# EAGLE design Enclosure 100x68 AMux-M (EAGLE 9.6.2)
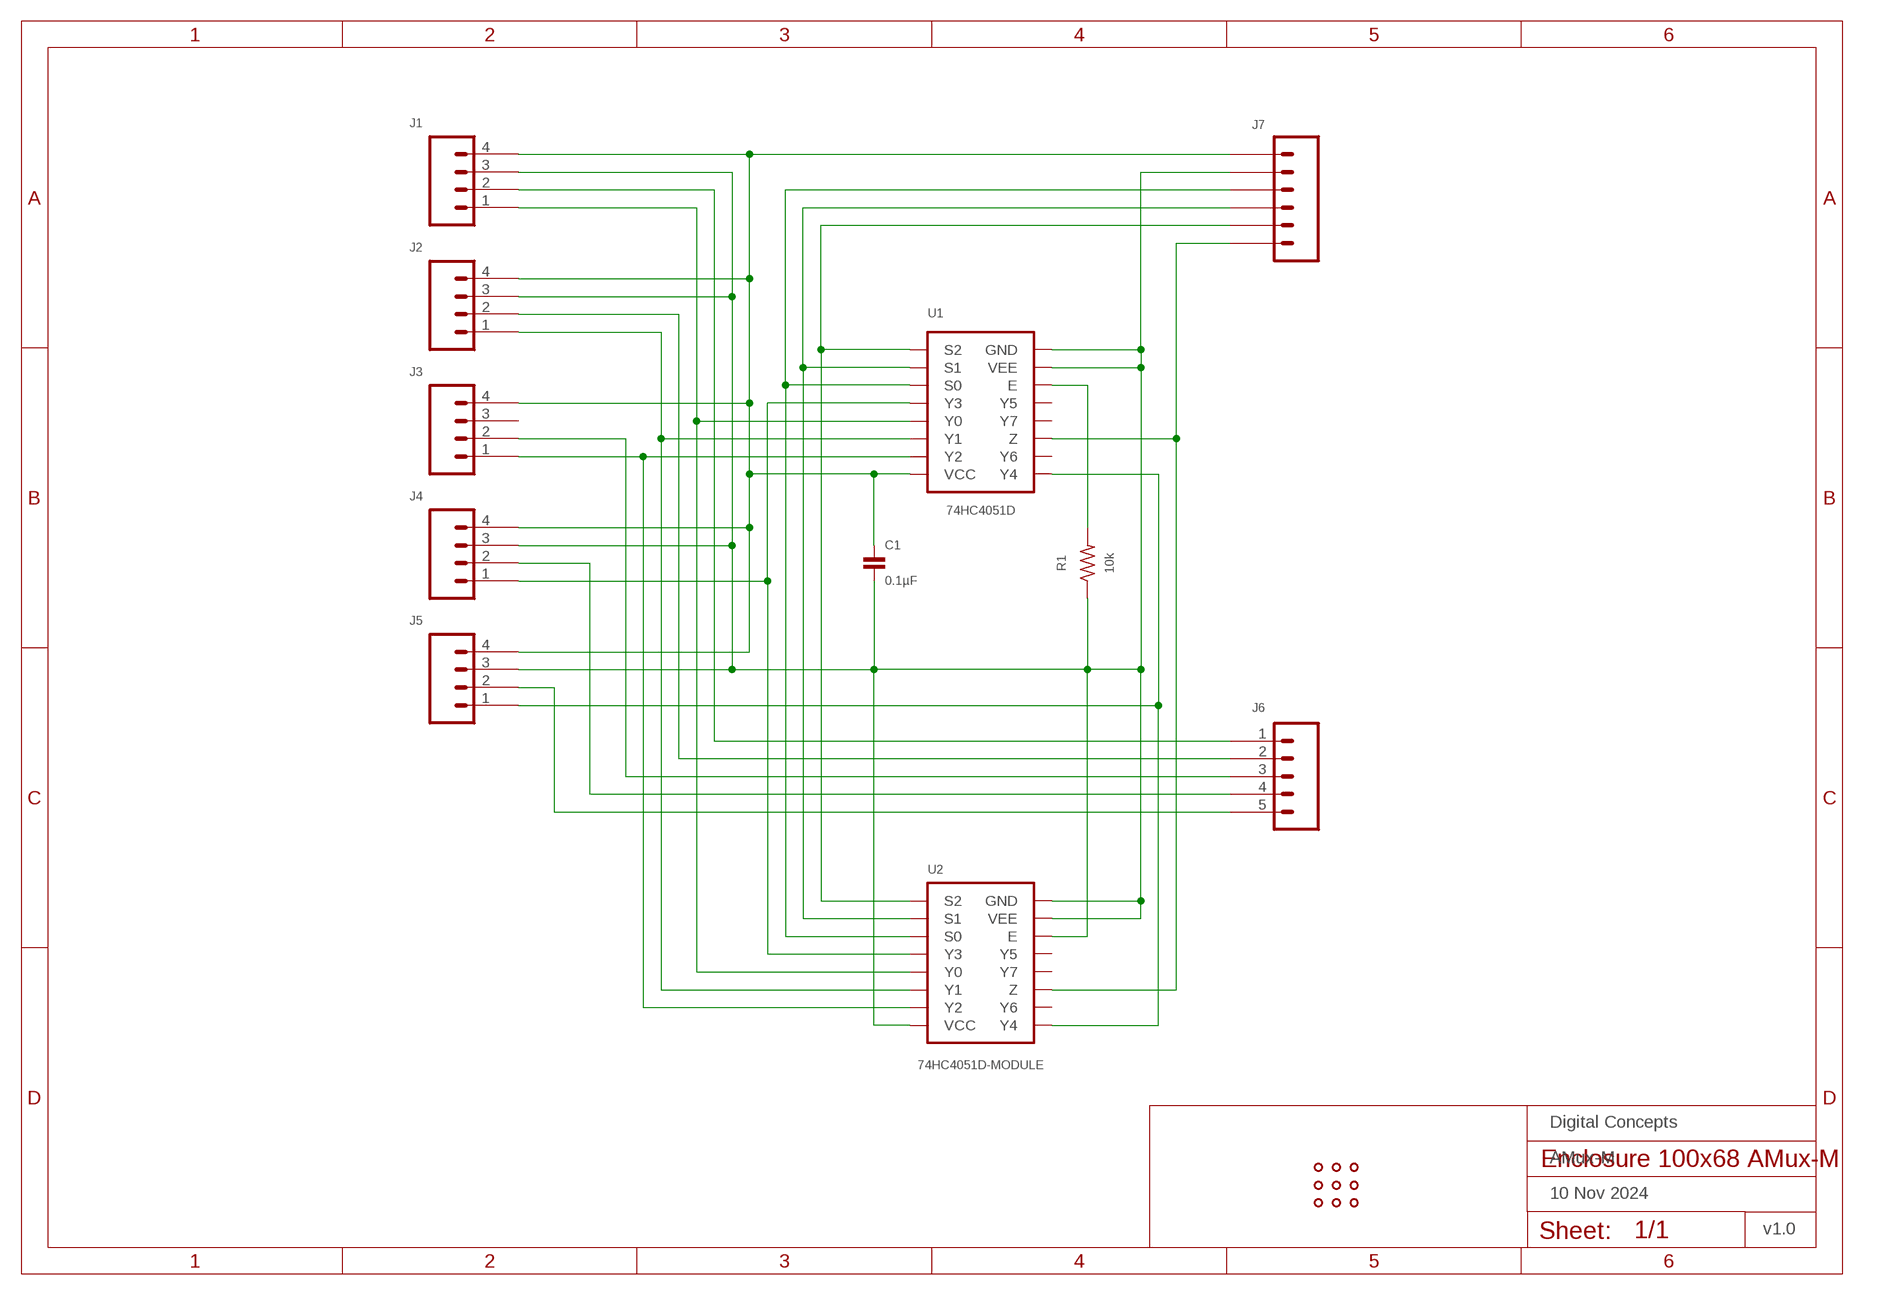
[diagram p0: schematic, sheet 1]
FRAME1 (A4L-LOC): DATE: 10 Nov 2024; OWNER: Digital Concepts; TITLE: AMux-M; VERSION: v1.0

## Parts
C1  0.1µF  CAPACITOR-0805  [C0805]
J1  HEADER-1X4-GENERIC  [CONN_04-GENERIC]
J2  HEADER-1X4-GENERIC  [CONN_04-GENERIC]
J3  HEADER-1X4-GENERIC  [CONN_04-GENERIC]
J4  HEADER-1X4-GENERIC  [CONN_04-GENERIC]
J5  HEADER-1X4-GENERIC  [CONN_04-GENERIC]
J6  JST-PH2.0-5-HORIZONTAL  [JST-PH2.0-5-HORIZONTAL]
J7  JST-PH2.0-6-HORIZONTAL  [JST-PH2.0-6-HORIZONTAL]
R1  10k  RESISTORR0805  [R0805]
U1  74HC4051D  [SOP16]
U2  74HC4051D-MODULE  [74HC4051D-MODULE]
U$1  PROTO-34X22-AMUX  [PROTO-34X22-AMUX]

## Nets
GND: C1.2 J1.3 J2.3 J4.3 J5.3 J7.2 R1.1 U1.7(VEE) U1.8(GND) U2.E U2.GND@L(GND) U2.GND@R(GND) U2.VCC@L(VCC) U2.VCC@R(VCC) U2.VEE@L(VEE) U2.VEE@R(VEE)
N$1: J4.1 U1.12(Y3) U2.Y3
N$2: J2.1 U1.14(Y1) U2.Y1
N$3: J1.1 U1.13(Y0) U2.Y0
N$4: J3.1 U1.15(Y2) U2.Y2
N$5: J5.1 U1.1(Y4) U2.Y4
N$6: J7.3 U1.11(S0) U2.S0
N$7: J7.4 U1.10(S1) U2.S1
N$8: R1.2 U1.6(E)
N$9: J7.6 U1.3(Z) U2.Z
N$13: J1.2 J6.1
N$16: J7.5 U1.9(S2) U2.S2
N$17: J2.2 J6.2
N$18: J3.2 J6.3
N$19: J4.2 J6.4
N$20: J5.2 J6.5
N$26: C1.1 J1.4 J2.4 J3.4 J4.4 J5.4 J7.1 U1.16(VCC)
Unconnected: J3.3 U1.2(Y6) U1.4(Y7) U1.5(Y5) U2.Y5 U2.Y6 U2.Y7

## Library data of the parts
C1 = digitalconcepts:CAPACITOR-0805: 0805 Capacitor
J1-J5 = digitalconcepts:HEADER-1X4-GENERIC: Single Row 4-Pin Header
J6 = digitalconcepts:JST-PH2.0-5-HORIZONTAL: PH2.0 5P Horizontal Connector
J7 = digitalconcepts:JST-PH2.0-6-HORIZONTAL: PH2.0 6P Horizontal Connector
R1 = digitalconcepts:RESISTOR: Resistor; SPICEPREFIX: R
U1 = digitalconcepts:74HC4051D: 74HC4051 8-Port Multiplexer SOP-16
U2 = digitalconcepts:74HC4051D-MODULE: 74HC4051 8-Port Analog Multiplexer Module
U$1 = digitalconcepts:PROTO-34X22-AMUX: 34 x 22 Analog Mux Prototyping board to fit an 100 x 68 enclosure

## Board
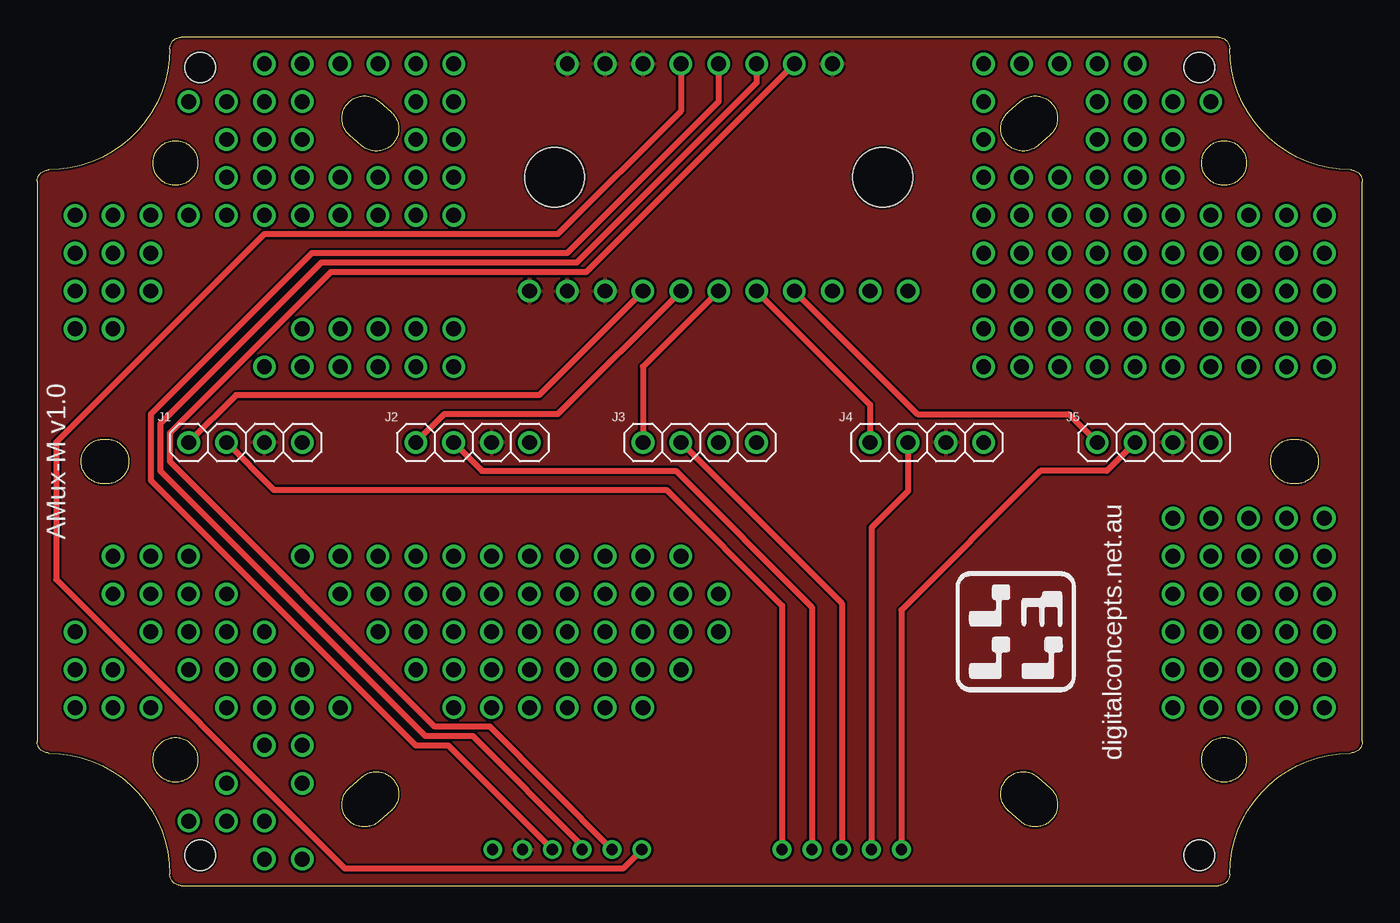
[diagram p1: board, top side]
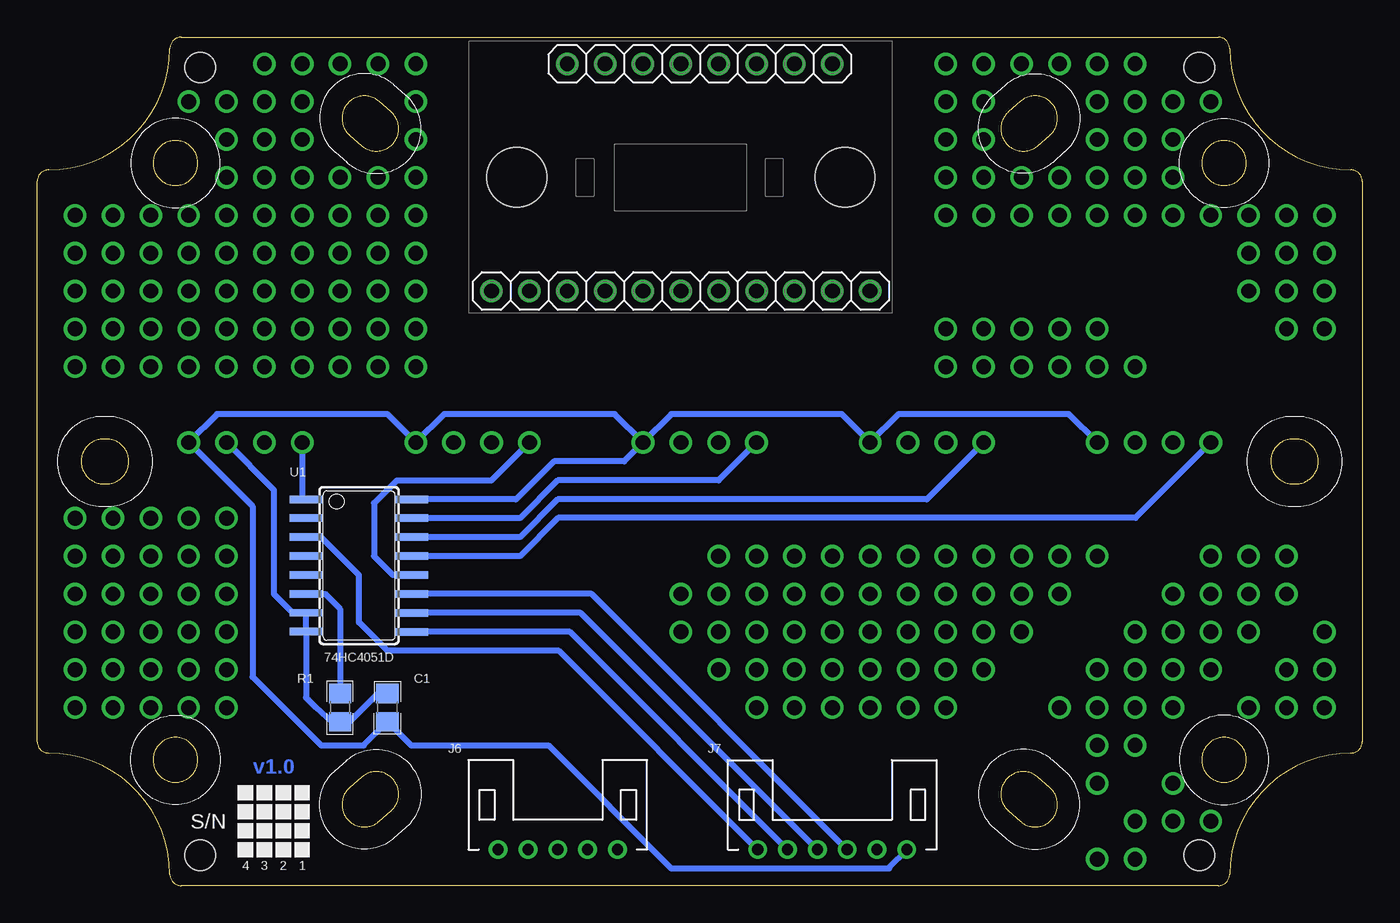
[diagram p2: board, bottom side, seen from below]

Size 88.9 x 56.9 mm. Coordinates in mm from the lower left corner, seen from the top.
Copper layers (1*16): Top 0.035mm / dielectric 1.5mm / Bottom 0.035mm
Design rules "default *": minimum track width 6mil, minimum drill 0.35mm, track to track 6mil, track to pad 6mil, pad to pad 6mil, via to via 6mil, smd to smd 6mil, copper to edge 6mil, drill to drill 6mil, minimum pad ring 10mil, minimum via ring 8mil, stop-mask expansion 4mil, vias tented up to drill 0mil, thermal gap 6mil

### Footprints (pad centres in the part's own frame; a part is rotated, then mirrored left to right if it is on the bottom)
C0805 = smd 1.3 x 1.5: 1 -0.95,0; 2 0.95,0
CONN_04-GENERIC = drill 1 pad 1.524: 1 0,0; 2 2.54,0; 3 5.08,0; 4 7.62,0
JST-PH2.0-5-HORIZONTAL = drill 0.75: 1 4,0; 2 2,0; 3 0,0; 4 -2,0; 5 -4,0
JST-PH2.0-6-HORIZONTAL = drill 0.75: 1 5,0; 2 3,0; 3 1,0; 4 -1,0; 5 -3,0; 6 -5,0
R0805 = smd 1.3 x 1.5: 1 -0.95,0; 2 0.95,0
SOP16 = smd 0.5 x 2.2: 1 -4.445,-3.55; 2 -3.185,-3.55; 3 -1.915,-3.55; 4 -0.645,-3.55; 5 0.635,-3.55; 6 1.895,-3.55; 7 3.165,-3.55; 8 4.435,-3.55; 9 4.445,3.55; 10 3.175,3.55; 11 1.905,3.55; 12 0.635,3.55; 13 -0.635,3.55; 14 -1.905,3.55; 15 -3.175,3.55; 16 -4.445,3.55
74HC4051D-MODULE = drill 1: E 0,5.08; GND@L 0,17.78; GND@R 15.24,20.32; S0 0,12.7; S1 0,10.16; S2 0,7.62; VCC@L 0,20.32; VCC@R 15.24,22.86; VEE@L 0,22.86; VEE@R 15.24,25.4; Y0 15.24,17.78; Y1 15.24,15.24; Y2 15.24,12.7; Y3 15.24,10.16; Y4 15.24,7.62; Y5 15.24,5.08; Y6 15.24,2.54; Y7 15.24,0; Z 0,15.24 | hole 4: 7.62,23.7; 7.62,1.7
PROTO-34X22-AMUX = drill 1: P01-05 -41.91,-16.51; P01-06 -41.91,-13.97; P01-07 -41.91,-11.43; P01-15 -41.91,8.89; P01-16 -41.91,11.43; P01-17 -41.91,13.97; P01-18 -41.91,16.51; P02-05 -39.37,-16.51; P02-06 -39.37,-13.97; P02-08 -39.37,-8.89; P02-09 -39.37,-6.35; P02-15 -39.37,8.89; P02-16 -39.37,11.43; P02-17 -39.37,13.97; P02-18 -39.37,16.51; P03-05 -36.83,-16.51; P03-07 -36.83,-11.43; P03-08 -36.83,-8.89; P03-09 -36.83,-6.35; P03-16 -36.83,11.43; P03-17 -36.83,13.97; P03-18 -36.83,16.51; P04-02 -34.29,-24.13; P04-06 -34.29,-13.97; P04-07 -34.29,-11.43; P04-08 -34.29,-8.89; P04-09 -34.29,-6.35; P04-18 -34.29,16.51; P04-21 -34.29,24.13; P05-02 -31.75,-24.13; P05-03 -31.75,-21.59; P05-05 -31.75,-16.51; P05-06 -31.75,-13.97; P05-07 -31.75,-11.43; P05-08 -31.75,-8.89; P05-18 -31.75,16.51; P05-19 -31.75,19.05; P05-20 -31.75,21.59; P05-21 -31.75,24.13; P06-01 -29.21,-26.67; P06-02 -29.21,-24.13; P06-04 -29.21,-19.05; P06-05 -29.21,-16.51; P06-06 -29.21,-13.97; P06-07 -29.21,-11.43; P06-14 -29.21,6.35; P06-18 -29.21,16.51; P06-19 -29.21,19.05; P06-20 -29.21,21.59; P06-21 -29.21,24.13; P06-22 -29.21,26.67; P07-01 -26.67,-26.67; P07-03 -26.67,-21.59; P07-04 -26.67,-19.05; P07-05 -26.67,-16.51; P07-06 -26.67,-13.97; P07-09 -26.67,-6.35; P07-14 -26.67,6.35; P07-15 -26.67,8.89; P07-18 -26.67,16.51; P07-19 -26.67,19.05; P07-20 -26.67,21.59; P07-21 -26.67,24.13; P07-22 -26.67,26.67; P08-05 -24.13,-16.51; P08-08 -24.13,-8.89; P08-09 -24.13,-6.35; P08-14 -24.13,6.35; P08-15 -24.13,8.89; P08-18 -24.13,16.51; P08-19 -24.13,19.05; P08-22 -24.13,26.67; P09-07 -21.59,-11.43; P09-08 -21.59,-8.89; P09-09 -21.59,-6.35; P09-14 -21.59,6.35; P09-15 -21.59,8.89; P09-18 -21.59,16.51; P09-19 -21.59,19.05; P09-22 -21.59,26.67; P10-06 -19.05,-13.97; P10-07 -19.05,-11.43; P10-08 -19.05,-8.89; P10-09 -19.05,-6.35; P10-14 -19.05,6.35; P10-15 -19.05,8.89; P10-18 -19.05,16.51; P10-19 -19.05,19.05; P10-20 -19.05,21.59; P10-21 -19.05,24.13; P10-22 -19.05,26.67; P11-05 -16.51,-16.51; P11-06 -16.51,-13.97; P11-07 -16.51,-11.43; P11-08 -16.51,-8.89; P11-09 -16.51,-6.35; P11-14 -16.51,6.35; P11-15 -16.51,8.89; P11-18 -16.51,16.51; P11-19 -16.51,19.05; P11-20 -16.51,21.59; P11-21 -16.51,24.13; P11-22 -16.51,26.67; P12-05 -13.97,-16.51; P12-06 -13.97,-13.97; P12-07 -13.97,-11.43; P12-08 -13.97,-8.89; P12-09 -13.97,-6.35; P13-05 -11.43,-16.51; P13-06 -11.43,-13.97; P13-07 -11.43,-11.43; P13-08 -11.43,-8.89; P13-09 -11.43,-6.35; P14-05 -8.89,-16.51; P14-06 -8.89,-13.97; P14-07 -8.89,-11.43; P14-08 -8.89,-8.89; P14-09 -8.89,-6.35; P15-05 -6.35,-16.51; P15-06 -6.35,-13.97; P15-07 -6.35,-11.43; P15-08 -6.35,-8.89; P15-09 -6.35,-6.35; P16-05 -3.81,-16.51; P16-06 -3.81,-13.97; P16-07 -3.81,-11.43; P16-08 -3.81,-8.89; P16-09 -3.81,-6.35; P17-06 -1.27,-13.97; P17-07 -1.27,-11.43; P17-08 -1.27,-8.89; P17-09 -1.27,-6.35; P18-07 1.27,-11.43; P18-08 1.27,-8.89; P25-14 19.05,6.35; P25-15 19.05,8.89; P25-16 19.05,11.43; P25-17 19.05,13.97; P25-18 19.05,16.51; P25-19 19.05,19.05; P25-20 19.05,21.59; P25-21 19.05,24.13; P25-22 19.05,26.67; P26-14 21.59,6.35; P26-15 21.59,8.89; P26-16 21.59,11.43; P26-17 21.59,13.97; P26-18 21.59,16.51; P26-19 21.59,19.05; P26-22 21.59,26.67; P27-14 24.13,6.35; P27-15 24.13,8.89; P27-16 24.13,11.43; P27-17 24.13,13.97; P27-18 24.13,16.51; P27-19 24.13,19.05; P27-22 24.13,26.67; P28-14 26.67,6.35; P28-15 26.67,8.89; P28-16 26.67,11.43; P28-17 26.67,13.97; P28-18 26.67,16.51; P28-19 26.67,19.05; P28-20 26.67,21.59; P28-21 26.67,24.13; P28-22 26.67,26.67; P29-14 29.21,6.35; P29-15 29.21,8.89; P29-16 29.21,11.43; P29-17 29.21,13.97; P29-18 29.21,16.51; P29-19 29.21,19.05; P29-20 29.21,21.59; P29-21 29.21,24.13; P29-22 29.21,26.67; P30-05 31.75,-16.51; P30-06 31.75,-13.97; P30-07 31.75,-11.43; P30-08 31.75,-8.89; P30-09 31.75,-6.35; P30-10 31.75,-3.81; P30-14 31.75,6.35; P30-15 31.75,8.89; P30-16 31.75,11.43; P30-17 31.75,13.97; P30-18 31.75,16.51; P30-19 31.75,19.05; P30-20 31.75,21.59; P30-21 31.75,24.13; P31-05 34.29,-16.51; P31-06 34.29,-13.97; P31-07 34.29,-11.43; P31-08 34.29,-8.89; P31-09 34.29,-6.35; P31-10 34.29,-3.81; P31-14 34.29,6.35; P31-15 34.29,8.89; P31-16 34.29,11.43; P31-17 34.29,13.97; P31-18 34.29,16.51; P31-21 34.29,24.13; P32-05 36.83,-16.51; P32-06 36.83,-13.97; P32-07 36.83,-11.43; P32-08 36.83,-8.89; P32-10 36.83,-3.81; P32-14 36.83,6.35; P32-15 36.83,8.89; P32-16 36.83,11.43; P32-17 36.83,13.97; P32-18 36.83,16.51; P33-05 39.37,-16.51; P33-06 39.37,-13.97; P33-07 39.37,-11.43; P33-08 39.37,-8.89; P33-10 39.37,-3.81; P33-14 39.37,6.35; P33-15 39.37,8.89; P33-16 39.37,11.43; P33-17 39.37,13.97; P33-18 39.37,16.51; P34-05 41.91,-16.51; P34-06 41.91,-13.97; P34-07 41.91,-11.43; P34-08 41.91,-8.89; P34-09 41.91,-6.35; P34-10 41.91,-3.81; P34-14 41.91,6.35; P34-15 41.91,8.89; P34-16 41.91,11.43; P34-17 41.91,13.97; P34-18 41.91,16.51; P303 36.83,-6.35; P304 39.37,-6.35 | hole 2.032: -33.528,26.416; 33.528,26.416; 33.528,-26.416; -33.528,-26.416

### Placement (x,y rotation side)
C1  65.41,11.94 90 bottom
J1  10.16,29.72 0 top
J2  25.4,29.72 0 top
J3  40.64,29.72 0 top
J4  55.88,29.72 0 top
J5  71.12,29.72 0 top
J6  53.98,2.41 0 bottom
J7  35.56,2.41 0 bottom
R1  68.58,11.94 90 bottom
U1  67.31,21.46 270 bottom
U2  58.42,55.12 270 bottom
U$1  44.45,28.45 0 top

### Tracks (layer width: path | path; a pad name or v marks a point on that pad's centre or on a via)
GND
  Bottom 0.406: C1.2 66.05,12.89 67.95,10.99 R1.1 69.16,10.99 70.23,11.96 70.86,12.6 U1.8 U1.7 71.76,18.3 73.03,19.57 73.03,26.54 J5.3
  pour Top: -0.63,57.66 89.54,57.66 89.54,-0.76 -0.63,-0.76
N$1
  Top 0.406: U2.Y3 55.88,32.26 J4.1
  Bottom 0.406: J4.1 58.42,27.18 64.77,27.18 66.3,25.65 66.3,22.1 65.03,20.83 U1.12
N$2
  Top 0.406: U2.Y1 34.93,31.62 27.31,31.62 J2.1
  Bottom 0.406: J2.1 29.21,25.91 53.98,25.91 56.52,23.37 U1.14
N$3
  Top 0.406: U2.Y0 33.66,32.89 13.34,32.89 J1.1
  Bottom 0.406: J1.1 15.22,24.66 53.96,24.66 56.52,22.1 U1.13
N$4
  Top 0.406: U2.Y2 40.64,34.8 J3.1
  Bottom 0.406: J3.1 43.18,27.18 53.98,27.18 56.52,24.64 U1.15
N$5
  Top 0.406: U2.Y4 59.06,31.62 69.22,31.62 J5.1
  Bottom 0.406: U1.1 71.12,25.91 J5.1
N$6
  Top 0.406: U2.S0 45.72,52.58 35.56,42.42 18.42,42.42 7.62,31.62 7.62,27.18 25.4,9.4 27.58,9.4 J7.3
  Bottom 0.406: U1.11 51.71,19.56 J7.3
N$7
  Top 0.406: U2.S1 48.26,53.85 36.2,41.78 19.05,41.78 8.26,30.99 8.26,27.81 26.04,10.03 29.21,10.03 36.56,2.68 J7.4
  Bottom 0.406: J7.4 52.44,18.29 U1.10
N$8
  Bottom 0.406: R1.2 68.58,18.56 69.59,19.57 U1.6
N$9
  Top 0.406: U2.Z 43.18,51.94 34.93,43.69 15.24,43.69 1.27,29.72 1.27,20.53 20.66,1.14 39.29,1.14 J7.6
  Bottom 0.406: J7.6 53.9,15.75 65.41,15.75 67.31,17.65 67.31,20.83 69.86,23.38 U1.3
N$13
  Top 0.406: J6.1 49.98,18.78 42.21,26.54 15.88,26.54 J1.2
N$16
  Top 0.406: U2.S2 36.83,41.15 19.69,41.15 8.89,30.35 8.89,28.45 26.67,10.67 30.38,10.67 J7.5
  Bottom 0.406: J7.5 53.17,17.02 U1.9
N$17
  Top 0.406: J6.2 51.98,18.68 42.84,27.81 29.85,27.81 J2.2
N$18
  Top 0.406: J6.3 53.98,18.92 J3.2
N$19
  Top 0.406: J6.4 55.98,24 58.42,26.45 J4.2
N$20
  Top 0.406: J6.5 57.98,18.48 67.31,27.81 71.76,27.81 J5.2
N$26
  Bottom 0.406: J1.4 19.69,31.62 31.12,31.62 J2.4 34.93,31.62 46.36,31.62 J3.4 | J3.4 50.17,31.62 61.59,31.62 J4.4 65.41,31.62 76.84,31.62 J5.4 74.46,25.43 74.46,14 69.85,9.4 67,9.4 C1.1 63.82,9.4 54.61,9.4 46.36,1.14 31.75,1.14 31.75,1.22 J7.1 | J3.4 49.53,28.45 54.24,28.45 56.78,25.91 U1.16

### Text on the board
Bottom: v1.0
tPlace: AMux-M v1.0 | digitalconcepts.net.au
bPlace: S/N | 1 | 2 | 3 | 4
